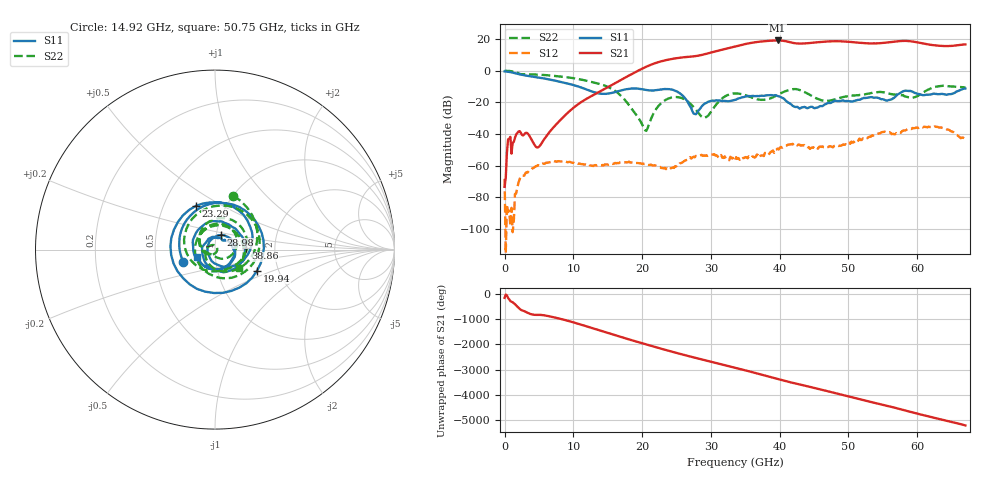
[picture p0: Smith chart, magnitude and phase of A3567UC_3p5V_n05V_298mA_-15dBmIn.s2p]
! MARKI MICROWAVE INC.
! Date:  4/20/2021
! Model Number:  A-3567UC
! Description:  2-port Small Signal S-parameter data for A-3567UC
! Frequency Range:  10 MHz to 67 GHz
! Port Configuration:  PORT 1: Input
!  PORT 2: Output
! Bias Condition: Vd = +3.5V, Vg = -0.5V, Id = 298mA
! A-3567UC s2p files are only valid for small signal conditions (below -10 dBm input power)
# Hz S  dB  R 50
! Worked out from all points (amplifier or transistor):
!   401 points, 10 MHz to 67 GHz, reference 50 ohm
!   highest |S21| = 19.2 dB at 39.7 GHz (marker M1)
!   |S21| within 3 dB of that: 34.25 GHz to 62.38 GHz (28.13 GHz wide, 58.2 % of centre)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
!   unconditionally stable (mu >= 1): 178.4 MHz to end of sweep
!   at 11.06 GHz: K = 2855.62, MAG = -18.1 dB, |S12| = -58.9 dB
!   at 33.51 GHz: K = 57.03, MAG = 15.6 dB, |S12| = -57.0 dB
!   at 67 GHz: K = 7.88, MAG = 17.4 dB, |S12| = -42.0 dB
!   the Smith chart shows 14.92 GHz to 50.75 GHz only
!   S11 on the Smith chart (normalised r, x): 14.92 GHz: 0.70, -0.10; 19.94 GHz: 1.55, -0.39; 23.29 GHz: 0.72, +0.38; 28.98 GHz: 1.05, +0.17; 38.86 GHz: 1.41, +0.02; 50.75 GHz: 0.81, -0.07
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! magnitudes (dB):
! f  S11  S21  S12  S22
! 10 MHz  -0.4  -73.3  -68.3  0.0
! 679.9 MHz  -0.7  -43.1  -88.4  -0.1
! 1.852 GHz  -1.9  -39.3  -73.9  -1.2
! 4.867 GHz  -4.2  -48.4  -59.6  -2.4
! 11.23 GHz  -10.7  -19.5  -59.0  -5.6
! 14.92 GHz  -14.5  -10.6  -59.1  -10.0
! 19.94 GHz  -11.6  1.2  -58.8  -33.3
! 20.78 GHz  -12.2  2.9  -59.3  -36.5
! 22.45 GHz  -12.0  5.6  -60.8  -21.9
! 23.29 GHz  -11.5  6.6  -61.3  -18.7
! 25.63 GHz  -14.7  8.4  -58.3  -17.1
! 27.64 GHz  -27.2  9.2  -54.6  -23.7
! 28.98 GHz  -21.1  10.4  -53.5  -29.7
! 33.51 GHz  -18.3  15.4  -57.0  -14.3
! 38.86 GHz  -15.4  19.1  -50.9  -17.1
! 39.7 GHz  -15.9  19.2  -49.2  -15.2
! 44.73 GHz  -22.8  17.7  -48.6  -16.0
! 50.75 GHz  -19.1  18.1  -44.8  -15.5
! 55.95 GHz  -18.4  18.0  -38.8  -14.5
! 59.46 GHz  -13.5  18.4  -36.3  -16.8
! 62.81 GHz  -14.6  16.0  -35.4  -9.9
! 67 GHz  -11.2  16.7  -42.0  -10.5
